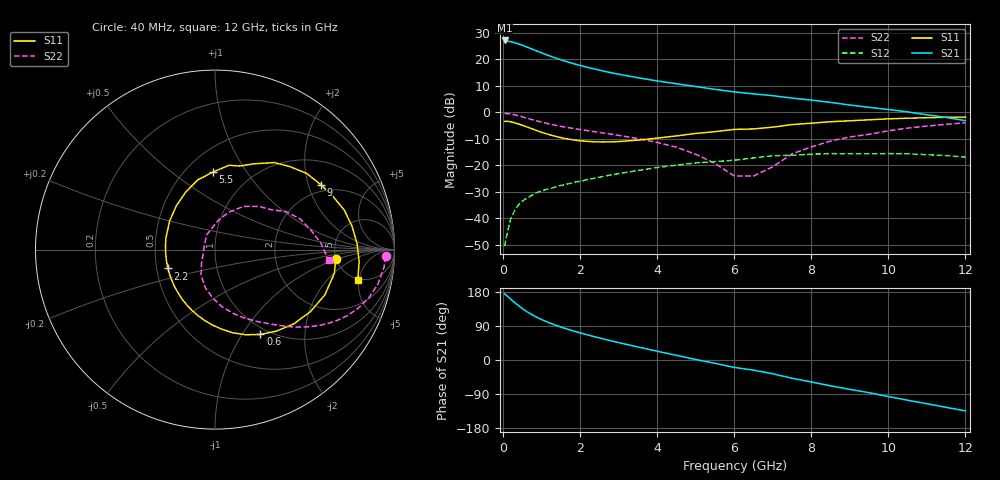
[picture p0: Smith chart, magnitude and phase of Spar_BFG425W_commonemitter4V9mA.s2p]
! Filename: 49bfg425.001
! BFG425W Field C1
! V1=8.315E-001V,V2=4.000E+000V, I1=9.911E-005A, I2=8.990E-003A
# GHz  S  MA  R 50
!  S11  S21  S12  S22
!Freq(GHz)  Mag  Ang  Mag  Ang  Mag  Ang  Mag  Ang
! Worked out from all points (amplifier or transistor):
!   44 points, 40 MHz to 12 GHz, reference 50 ohm
!   highest |S21| = 27.1 dB at 40 MHz (marker M1)
!   |S21| within 3 dB of that: start of sweep to 708.9 MHz
!   unconditionally stable (mu >= 1): 1.963 GHz to end of sweep
!   at 700 MHz: K = 0.52, MSG = 27.9 dB, |S12| = -31.7 dB
!   at 2.4 GHz: K = 1.09, MAG = 18.7 dB, |S12| = -24.7 dB
!   at 12 GHz: K = 1.41, MAG = 3.1 dB, |S12| = -16.9 dB
!   S11 on the Smith chart (normalised r, x): 40 MHz: 4.96, -0.95; 600 MHz: 0.91, -1.21; 2.2 GHz: 0.57, -0.13; 5.5 GHz: 0.67, +0.71; 9 GHz: 1.75, +2.42; 12 GHz: 4.82, -4.80
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0.04  0.675 -4.4  22.6 174.7  0.003 46.3  0.951 -2.3
0.2  0.662 -22.4  21.4 160.2  0.01 71.0  0.928 -11.9
0.3  0.634 -33.1  20.5 151.7  0.014 68.8  0.898 -17.4
0.4  0.603 -43.3  19.48 143.5  0.018 64.9  0.862 -22.3
0.5  0.569 -52.9  18.39 135.5  0.021 61.6  0.823 -26.6
0.6  0.536 -61.8  17.2 128.8  0.024 58.9  0.784 -30.4
0.8  0.474 -77.9  15.05 116.9  0.029 54.2  0.712 -36.5
0.9  0.445 -85.1  14.08 111.6  0.031 52.4  0.681 -39.1
1.2  0.379 -104.8  11.61 98.1  0.036 48.6  0.603 -45.5
1.4  0.347 -116.6  10.32 90.5  0.04 46.9  0.562 -49.0
1.6  0.322 -127.9  9.265 83.7  0.043 45.5  0.528 -52.2
1.9  0.296 -143.6  7.993 74.4  0.049 43.4  0.486 -56.8
2.2  0.283 -158.2  7.006 66.0  0.054 41.3  0.45 -61.5
3  0.281 166.5  5.221 45.9  0.07 34.6  0.368 -74.3
3.5  0.299 147.8  4.482 34.4  0.08 29.4  0.32 -83.1
4.5  0.359 117.2  3.447 12.4  0.101 16.8  0.22 -103.9
5.5  0.432 91.6  2.708 -8.8  0.118 2.5  0.109 -133.6
6.5  0.486 73.4  2.224 -26.8  0.138 -8.3  0.063 161.1
8.5  0.664 39.7  1.536 -68.2  0.167 -44.9  0.288 56.7
9  0.692 31.5  1.372 -77.5  0.165 -53.2  0.343 44.5
10.5  0.774 9.9  1.018 -106.2  0.165 -80.5  0.504 19.9
12  0.813 -12.0  0.696 -134.3  0.143 -111.3  0.636 -5.4
